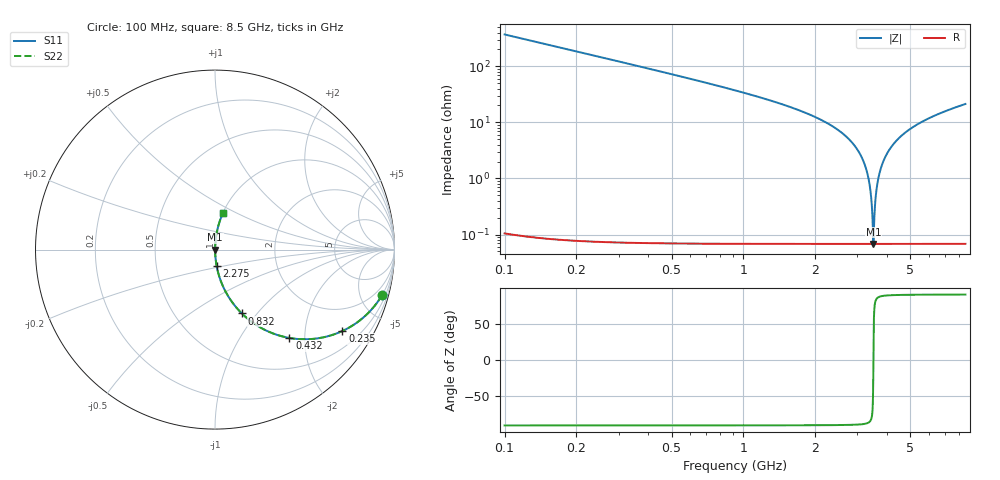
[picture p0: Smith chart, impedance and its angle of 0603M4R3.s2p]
! Created Wed Apr 18 15:47:24 2012
# hz S ma R 50
! 2 Port Network Data from SP1.SP block
! freq  magS11  angS11  magS21  angS21  magS12  angS12  magS22  angS22
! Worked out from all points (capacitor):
!   8401 points, 100 MHz to 8.5 GHz, reference 50 ohm
!   read as one part in series: C = 4.31 pF near 142 MHz
!   lowest |Z| = 68.2 mohm at 3.501 GHz (marker M1)
!   series resonance near 3.501 GHz, so ESL is about 480 pH
!   S11 on the Smith chart (normalised r, x): 100 MHz: 1.00, -7.38; 235 MHz: 1.00, -3.13; 432 MHz: 1.00, -1.68; 832 MHz: 1.00, -0.84; 2.275 GHz: 1.00, -0.19; 8.5 GHz: 1.00, +0.43
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1e8  0.9651 -15.2  0.2616 74.8  0.2616 74.8  0.9651 -15.2
2.35e8  0.8424 -32.6  0.5385 57.4  0.5385 57.4  0.8424 -32.6
4.32e8  0.6437 -49.9  0.7647 40.1  0.7647 40.1  0.6437 -49.9
8.32e8  0.386 -67.2  0.9218 22.7  0.9218 22.7  0.386 -67.2
1.5e9  0.1969 -78.4  0.9797 11.4  0.9797 11.4  0.1969 -78.4
2.275e9  0.09333 -84.2  0.995 5.4  0.995 5.4  0.09333 -84.2
2.9e9  0.03994 -86.7  0.9985 2.3  0.9985 2.3  0.03994 -86.7
3.148e9  0.02248 -87.0  0.9991 1.3  0.9991 1.3  0.02248 -87.0
3.315e9  0.01156 -86.0  0.9993 0.7  0.9993 0.7  0.01156 -86.0
3.407e9  0.005803 -82.9  0.9993 0.3  0.9993 0.3  0.005803 -82.9
3.475e9  0.001735 -66.8  0.9993 0.1  0.9993 0.1  0.001735 -66.8
3.501e9  0.0006819 -2.0  0.9993 0.0  0.9993 0.0  0.0006819 -2.0
3.527e9  0.001681 66.0  0.9993 -0.1  0.9993 -0.1  0.001681 66.0
3.568e9  0.004031 80.0  0.9993 -0.2  0.9993 -0.2  0.004031 80.0
3.605e9  0.006187 83.3  0.9993 -0.4  0.9993 -0.4  0.006187 83.3
3.728e9  0.01325 86.3  0.9992 -0.8  0.9992 -0.8  0.01325 86.3
3.955e9  0.02575 87.0  0.999 -1.5  0.999 -1.5  0.02575 87.0
4.3e9  0.04359 86.6  0.9984 -2.5  0.9984 -2.5  0.04359 86.6
4.88e9  0.07113 85.4  0.9968 -4.1  0.9968 -4.1  0.07113 85.4
5.7e9  0.1063 83.5  0.9937 -6.1  0.9937 -6.1  0.1063 83.5
7.1e9  0.1598 80.6  0.9865 -9.2  0.9865 -9.2  0.1598 80.6
8.5e9  0.2081 77.8  0.9774 -12.0  0.9774 -12.0  0.2081 77.8
